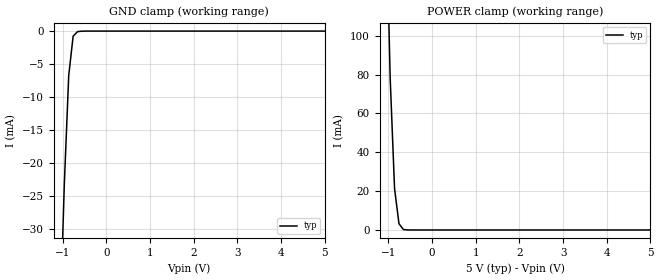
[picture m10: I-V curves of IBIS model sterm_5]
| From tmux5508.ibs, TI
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| sterm_5
[Model]   sterm_5
Model_type   Terminator
|   typ   min   max
C_comp   2.533030e-12   NA   NA
[Voltage Range]   5   NA   NA
[Temperature Range]   27   NA   NA
[Power Clamp Reference]   5   NA   NA
[GND Clamp Reference]   0   NA   NA
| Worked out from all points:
|   GND clamp passes 1 mA (typ) near -0.76 V on its own axis
|   POWER clamp passes 1 mA (typ) near -0.68 V on its own axis
[GND Clamp]
|   Voltage   I(typ)   I(min)   I(max)
-5V       -2.839A    NA         NA
-1.061V   -45mA      NA         NA
-959.6mV  -23.25mA   NA         NA
-858.6mV  -6.731mA   NA         NA
-757.6mV  -768.2uA   NA         NA
-656.6mV  -81.6uA    NA         NA
5V        469.4pA    NA         NA
[POWER Clamp]
|   Voltage   I(typ)   I(min)   I(max)
-5V       6.669A     NA         NA
-1.061V   177.1mA    NA         NA
-959.6mV  78.76mA    NA         NA
-858.6mV  21.38mA    NA         NA
-757.6mV  3.235mA    NA         NA
-656.6mV  232.6uA    NA         NA
5V        -576.6pA   NA         NA
